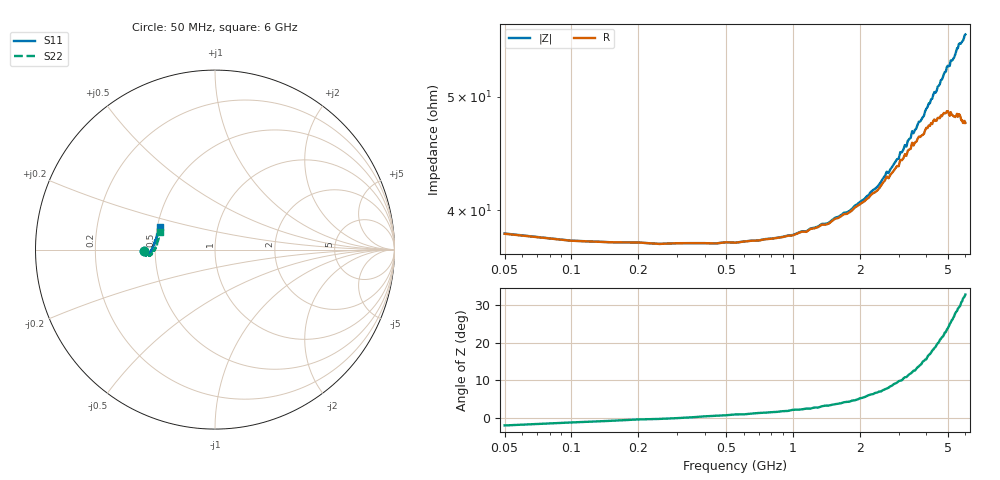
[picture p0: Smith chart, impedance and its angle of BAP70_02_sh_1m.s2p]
!	Created	by	janssen	on	Thu	Dec	12	13:21:33	MET	2002
#	HZ	S	MA	R	50
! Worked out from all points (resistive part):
!   120 points, 50 MHz to 6 GHz, reference 50 ohm
!   read as one part in shunt: R = 38.2 ohm at 50 MHz
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5e7  0.3957 -178.8  0.6054 -0.7  0.6039 -0.8  0.3965 -178.8
2.5e8  0.3997 -178.9  0.5992 0.4  0.5989 0.3  0.3996 -178.8
1.05e9  0.3964 -177.0  0.6048 3.1  0.6036 3.0  0.3935 -176.6
2.05e9  0.3818 -176.0  0.6219 5.8  0.6189 5.6  0.3798 -174.6
2.85e9  0.3691 -176.7  0.6423 7.6  0.6369 7.4  0.3621 -175.3
2.9e9  0.3666 -176.8  0.6417 7.7  0.6374 7.6  0.3578 -175.0
3e9  0.3653 -177.3  0.6446 7.9  0.6424 7.6  0.36 -175.5
3.05e9  0.3579 -177.8  0.6451 7.7  0.6408 7.8  0.3536 -175.6
3.1e9  0.3633 -177.2  0.6489 7.9  0.643 7.9  0.3575 -175.6
3.55e9  0.355 -178.9  0.6614 8.7  0.6561 8.6  0.3461 -177.2
4.05e9  0.3468 177.1  0.6765 9.3  0.6707 9.5  0.337 -179.8
4.3e9  0.3394 175.6  0.6832 9.6  0.6782 9.6  0.3327 177.9
4.35e9  0.3395 174.7  0.6856 9.8  0.6804 9.9  0.332 178.6
4.7e9  0.3389 171.7  0.6959 10.0  0.6861 10.1  0.3261 174.8
5e9  0.3313 168.8  0.7038 10.1  0.6985 10.5  0.3235 172.4
5.05e9  0.3345 168.4  0.704 10.2  0.698 10.5  0.3207 171.8
5.1e9  0.3336 167.5  0.7053 10.3  0.7011 10.5  0.324 171.2
5.5e9  0.3281 163.0  0.718 10.4  0.7122 10.8  0.3212 167.4
5.7e9  0.3321 161.5  0.7238 10.5  0.7162 10.9  0.3205 165.1
5.8e9  0.3285 159.9  0.7235 10.6  0.7191 11.0  0.3196 164.1
5.85e9  0.3328 158.7  0.7261 10.5  0.7203 11.0  0.3193 163.4
6e9  0.33 157.5  0.7301 10.5  0.727 11.1  0.3201 162.1
